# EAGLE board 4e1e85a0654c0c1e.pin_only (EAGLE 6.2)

Size 38 x 28.51 mm. Coordinates in mm from the lower left corner, seen from the top.
Outline: 0,4 0,25 arc-90 4,28.5 34,28.5 arc-90 38,24.5 38,4 arc-90 34,0 4,0 arc-90 0,4
Copper layers (1*16): Top 0.035mm / dielectric 1.5mm / Bottom 0.035mm
Design rules: minimum track width 8mil, minimum drill 0.4mm, track to track 8mil, track to pad 8mil, pad to pad 8mil, via to via 8mil, smd to smd 8mil, copper to edge 20mil, drill to drill 8mil, minimum pad ring 8mil, minimum via ring 10mil, stop-mask expansion 3mil, vias tented up to drill 20mil, thermal gap 8mil

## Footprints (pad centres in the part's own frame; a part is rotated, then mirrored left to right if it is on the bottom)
0805 = smd 1.3 x 1.5: 1 -0.95,0; 2 0.95,0
SOD-323 = smd 0.8 x 0.8: A 1.2,0; C -1.2,0
FIDUCIAL_1MM = smd 1 x 1: 1 0,0
1X08_ROUND_70 = drill 1 pad 1.778: 1 -8.89,0; 2 -6.35,0; 3 -3.81,0; 4 -1.27,0; 5 1.27,0; 6 3.81,0; 7 6.35,0; 8 8.89,0
SOT23-WIDE = smd 1 x 1.27: 1 -0.95,-1; 2 0.95,-1; 3 0,1
SOLDERJUMPER_REFLOW_NOPASTE = smd 1.168 x 1.6: 1 -0.762,0; 2 0.762,0
UG-2864HSWEG01_0.96IN_WRAPAROUND = smd 0.35 x 2.2 bottom: 1 -10.15,-1.2; 2 -9.45,-1.2; 3 -8.75,-1.2; 4 -8.05,-1.2; 5 -7.35,-1.2; 6 -6.65,-1.2; 7 -5.95,-1.2; 8 -5.25,-1.2; 9 -4.55,-1.2; 10 -3.85,-1.2; 11 -3.15,-1.2; 12 -2.45,-1.2; 13 -1.75,-1.2; 14 -1.05,-1.2; 15 -0.35,-1.2; 16 0.35,-1.2; 17 1.05,-1.2; 18 1.75,-1.2; 19 2.45,-1.2; 20 3.15,-1.2; 21 3.85,-1.2; 22 4.55,-1.2; 23 5.25,-1.2; 24 5.95,-1.2; 25 6.65,-1.2; 26 7.35,-1.2; 27 8.05,-1.2; 28 8.75,-1.2; 29 9.45,-1.2; 30 10.15,-1.2 | hole 0.4: -8,-5.45; 8,-5.45
SOT23-5 = smd 0.55 x 1.2: 1 -0.95,-1.3; 2 0,-1.3; 3 0.95,-1.3; 4 0.95,1.3; 5 -0.95,1.3
MOUNTINGHOLE_2.5_PLATED = drill 2.5 pad 3.2: P$1 0,0

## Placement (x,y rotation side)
C1  10uF  [0805]  27.91,20.88 90 bottom
C2  10uF  [0805]  23.66,14.64 180 bottom
C3  1uF  [0805]  3.11,6.62 0 bottom
C4  1uF  [0805]  3.11,8.75 180 bottom
C5  10uF  [0805]  29.44,11.53 270 bottom
C6  1uF  [0805]  2.98,11.28 0 bottom
C7  1uF  [0805]  2.98,13.44 0 bottom
C8  2.2uF/16V  [0805]  27.15,11.53 270 bottom
D1  1N4148  [SOD-323]  20.3,21.7 270 bottom
D2  1N4148  [SOD-323]  17.76,21.7 270 bottom
D3  1N4148  [SOD-323]  15.22,21.7 270 bottom
FID1  FIDUCIAL""  [FIDUCIAL_1MM]  31.73,25.36 0 bottom
FID2  FIDUCIAL""  [FIDUCIAL_1MM]  6.43,3.02 0 bottom
JP1  [1X08_ROUND_70]  19,25.43 0 top
Q1  BSS138  [SOT23-WIDE]  3.2,16.23 90 bottom
Q2  BSS138  [SOT23-WIDE]  3.16,21.09 90 bottom
R2  10K  [0805]  16.1,10.66 0 bottom
R3  390K  [0805]  24.61,11.53 270 bottom
R4  10K  [0805]  20.35,15.64 270 bottom
R5  10K  [0805]  17.75,15.64 270 bottom
R6  10K  [0805]  15.24,15.64 270 bottom
R11  10K  [0805]  9.53,14.36 90 bottom
R12  10K  [0805]  7.34,21.45 270 bottom
R13  10K  [0805]  7.34,14.36 90 bottom
R14  10K  [0805]  9.63,21.45 90 bottom
SJ1  [SOLDERJUMPER_REFLOW_NOPASTE]  34.5,11.99 0 bottom
SJ2  [SOLDERJUMPER_REFLOW_NOPASTE]  34.5,7.91 0 bottom
U1  UG-2864HSWEG01  [UG-2864HSWEG01_0.96IN_WRAPAROUND]  19.05,7.54 0 top
U2  [SOT23-5]  24.17,20.83 180 bottom
U$3  [ADAFRUIT_5MM]  35.56,19.05 0 bottom
U$23  MOUNTINGHOLE2.5  [MOUNTINGHOLE_2.5_PLATED]  35,25.5 0 top
U$24  MOUNTINGHOLE2.5  [MOUNTINGHOLE_2.5_PLATED]  3,3 0 top
U$25  MOUNTINGHOLE2.5  [MOUNTINGHOLE_2.5_PLATED]  35,3 0 top
U$26  MOUNTINGHOLE2.5  [MOUNTINGHOLE_2.5_PLATED]  3,25.5 0 top
U$27  [ADAFRUIT_2.5MM]  29.96,25.95 270 top
U$28  [LOGIC_5VREADY_5MM]  32.75,5.25 0 top

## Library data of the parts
C1-C8 D1-D3 FID1 FID2 JP1 Q1 Q2 R2-R6 R11-R14 SJ1 SJ2 U1 U2 U$3 U$23-U$28 = microbuilder

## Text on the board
tPlace: Data | SA0 | CS | Vin | Clk | DC | Rst | 3v3 | Gnd | v2.1
bPlace: SSD1306 0.96" 128x64 OLED | For I2C | Close | SJ1/2 | SJ1 | SJ2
